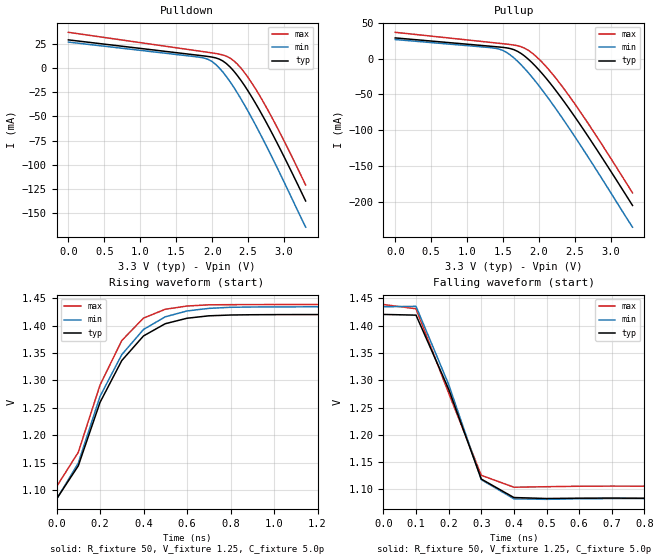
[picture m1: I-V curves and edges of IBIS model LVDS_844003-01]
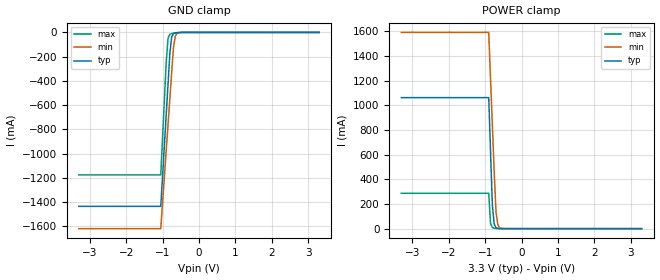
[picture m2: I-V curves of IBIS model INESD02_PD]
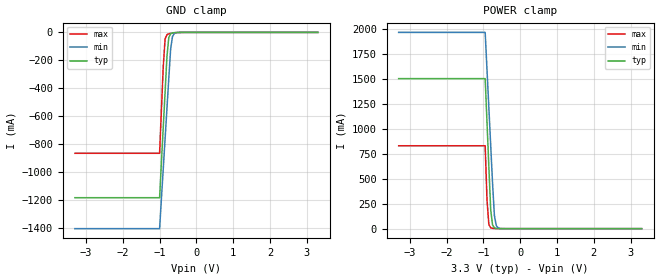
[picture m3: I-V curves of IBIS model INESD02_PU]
|   This file is an IBIS representation of the   |
|   Integrated Device Technology, Inc.   |
|   ICS844003-01   |
[IBIS Ver]   4.0
[File name]   844003-01_3v3.ibs
[File Rev]   1.0
[Date]   Sep 5 2007  | Last modified
|   Sep 5 2007  | Generated
[Source] Originated at Integrated Device Technology, Inc.
[Disclaimer]
IDT hereby grants the user of this IBIS model a non-exclusive,
nontransferable license to use this IBIS model under the following terms.
Before using this IBIS model, the user should read this license.
If the user does not accept these terms,  the IBIS model should be
returned to IDT within 30 days.
   The user is granted this license only to use the IBIS model and
is not granted rights to sell, load, rent, lease or license the IBIS
model in whole or in part, or in modified form to anyone other than
user. User may modify the IBIS model to suit its specific
applications but rights to derivative works and such modifications
shall belong to IDT.
   This IBIS model is provided on an "AS IS" basis and IDT makes
absolutely no warranty with respect to the information contained
herein. IDT DISCLAIMS AND CUSTOMER WAIVES ALL WARRANTIES, EXPRESS
OR IMPLIED, INCLUDING WARRANTIES OF MERCHANTABILITY OR FITNESS FOR
A PARTICULAR PURPOSE. The entire risk as to quality and performance
is with the Customer. ACCORDINGLY, IN NO EVENT SHALL THE COMPANY BE
LIABLE FOR ANY DAMAGES, WHETHER IN CONTRACT OR TORT,INCLUDING ANY
LOST PROFITS OR OTHER INCIDENTAL, CONSEQUENTIAL, EXEMPLARY, OR
PUNITIVE DAMAGES ARISING OUT OF THE USE OR APPLICATION OF THE IBIS
model provided in this package. Further, IDT reserves the right to
make changes without notice to any product herein to improve
reliability, function, or design. IDT does not convey any license
under patent rights or any other intellectual property rights,
including those of third parties.
   IDT is not obligated to provide maintenance or support
for the licensed IBIS model.
[Copyright]   Copyright 2007 by Integrated Device Technology, Inc.
[Component]   ICS844003BG-01
[Manufacturer] Integrated Device Technology, Inc.
[Package]
|TSSOP 24 Lead
|   typ   min   max
R_pkg   60.65m   52.4m   68.9m
L_pkg   1.989nH   1.431nH   2.547nH
C_pkg   0.314pF   0.254pF   0.374pF
[Pin] signal_name  model_name   R_pin   L_pin   C_pin
1   DIV_SELB0   INESD02_PU   68.9m   2.547n   0.374p
2   VCO_SEL   INESD02_PU   65.6m   2.323n   0.350p
3   MR   INESD02_PD   62.3m   2.100n   0.326p
4   VDDO_A   POWER   59.0m   1.877n   0.302p
5   QA0   LVDS_844003-01   55.7m   1.654n   0.278p
6   nQA0   LVDS_844003-01   52.4m   1.431n   0.254p
7   OEB   INESD02_PU   52.4m   1.431n   0.254p
8   OEA   INESD02_PU   55.7m   1.654n   0.278p
9   FB_DIV   INESD02_PD   59.0m   1.877n   0.302p
10   VDDA   POWER   62.3m   2.100n   0.326p
11   VDD   POWER   65.6m   2.323n   0.350p
12   DIV_SELA0   INESD02_PU   68.9m   2.547n   0.374p
13   DIV_SELA1   INESD02_PU   68.9m   2.547n   0.374p
14   GND   GND   65.6m   2.323n   0.350p
|15  XTAL_OUT   62.3m   2.100n   0.326p
|16  XTAL_IN   59.0m   1.877n   0.302p
17   REF_CLK   INESD02_PD   55.7m   1.654n   0.278p
18   XTAL_SEL   INESD02_PU   52.4m   1.431n   0.254p
19   nQB1   LVDS_844003-01   52.4m   1.431n   0.254p
20   QB1   LVDS_844003-01   55.7m   1.654n   0.278p
21   nQB0   LVDS_844003-01   59.0m   1.877n   0.302p
22   QB0   LVDS_844003-01   62.3m   2.100n   0.326p
23   VDDO_B   POWER   65.6m   2.323n   0.350p
24   DIV_SELB1   INESD02_PU   68.9m   2.547n   0.374p
[Diff Pin]  inv_pin  vdiff tdelay_typ tdelay_min  tdelay_max
5   6   NA   0  0  0
20   19   NA   0  0  0
22   21   NA   0  0  0
| Models and submodels in the file (3): LVDS_844003-01 (Output_ECL), INESD02_PD (Input), INESD02_PU (Input)
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[Model]   LVDS_844003-01
Model_type   Output_ECL
Polarity   Non-Inverting
|   onlvds01_lvds03_vrlvds06_abiasoff01_3v3_8402010i
|   typ   min   max
C_comp   2pF   1.5pF   2.5pF
Vmeas = 1.25V
Rref = 50
Vref = 1.25V
|   typ   min   max
[Voltage range]   3.3V   3.135V   3.465V
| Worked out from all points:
|   rising waveform, R_fixture 50, V_fixture 1.25, C_fixture 5.0p: 20-80 % time 231ps typ, 234ps min, 196ps max; typ from 1.08 V to 1.42 V
|   falling waveform, R_fixture 50, V_fixture 1.25, C_fixture 5.0p: 20-80 % time 132ps typ, 130ps min, 131ps max; typ from 1.42 V to 1.08 V
[pulldown]
|Voltage   I (typ)   I (min)   I (max)
0V        29.08mA    26.8mA     36.89mA
1.8V      13.22mA    11.37mA    17.73mA
1.9V      12.32mA    10.03mA    16.66mA
2V        11.24mA    6.613mA    15.58mA
2.15V     7.191mA    -4.325mA   13.43mA
2.25V     965.3uA    -14.33mA   10.19mA
2.35V     -7.741mA   -25.77mA   4.035mA
2.5V      -23.89mA   -44.84mA   -9.868mA
2.65V     -42.52mA   -65.56mA   -27.29mA
2.85V     -69.92mA   -94.93mA   -53.84mA
3.05V     -99.22mA   -125.7mA   -82.8mA
3.3V      -137.5mA   -164.6mA   -121mA
[pullup]
|Voltage   I (typ)   I (min)   I (max)
0V        29.08mA    26.8mA     36.89mA
1.35V     17.18mA    15.14mA    22.52mA
1.5V      15.75mA    11.38mA    20.91mA
1.6V      14.13mA    5.181mA    19.77mA
1.75V     7.285mA    -8.508mA   16.68mA
1.9V      -5.36mA    -25.52mA   8.171mA
2.05V     -21.61mA   -44.7mA    -5.816mA
2.2V      -40.2mA    -65.36mA   -23.15mA
2.4V      -67.42mA   -94.5mA    -49.51mA
2.65V     -104mA     -132.6mA   -85.74mA
2.95V     -150.1mA   -180mA     -132mA
3.3V      -205.5mA   -235.9mA   -187.9mA
[Ramp]
|   typ   min   max
dV/dt_r   0.24/0.3n   0.24/0.35n   0.24/0.25n
dV/dt_f   0.24/0.3n   0.24/0.35n   0.24/0.25n
[Rising Waveform]
R_fixture = 50
V_fixture = 1.25
V_fixture_max = 1.28
V_fixture_min = 1.22
C_fixture = 5.0p
| Time   typ   min   max
0s        1.083V     1.083V     1.106V
100ps     1.144V     1.149V     1.169V
200ps     1.26V      1.271V     1.292V
300ps     1.336V     1.347V     1.373V
400ps     1.381V     1.393V     1.414V
500ps     1.404V     1.416V     1.43V
600ps     1.414V     1.427V     1.436V
800ps     1.42V      1.434V     1.438V
1ns       1.42V      1.435V     1.439V
5ns       1.421V     1.435V     1.439V
[Falling Waveform]
R_fixture = 50
V_fixture = 1.25
V_fixture_max = 1.28
V_fixture_min = 1.22
C_fixture = 5.0p
| Time   typ   min   max
0s        1.421V     1.435V     1.439V
100ps     1.419V     1.435V     1.431V
200ps     1.284V     1.292V     1.277V
300ps     1.119V     1.118V     1.126V
400ps     1.085V     1.083V     1.104V
500ps     1.083V     1.082V     1.105V
700ps     1.084V     1.083V     1.106V
5ns       1.083V     1.083V     1.106V
[Model]   INESD02_PD
Model_type   Input
Polarity   Non-Inverting
Vinl = 0.80V
Vinh = 2.0V
|   typ   min   max
C_comp   2pF   1.5pF   2.5pF
|   typ   min   max
[Voltage range]  3.3V   3.15V   3.45V
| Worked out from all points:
|   GND clamp passes 1 mA (typ) near -0.56 V on its own axis
|   POWER clamp passes 1 mA (typ) near -0.61 V on its own axis
[GND_clamp]
|Voltage   I(typ)   I(min)   I(max)
-3.3V     -1.436A    -1.62A     -1.176A
-1.05V    -1.436A    -1.62A     -1.176A
-900mV    -678.5mA   -975.1mA   -244mA
-850mV    -426.1mA   -760.1mA   -46.85mA
-800mV    -173.9mA   -545.4mA   -16.11mA
-750mV    -36.96mA   -330.7mA   -9.916mA
-700mV    -9.696mA   -120.2mA   -7.056mA
-650mV    -3.545mA   -29.7mA    -4.857mA
-600mV    -1.629mA   -7.52mA    -3.049mA
-400mV    -52.81uA   -52.52uA   -108.7uA
3.3V      71.13uA    77.43uA    62.11uA
[POWER_clamp]
|Voltage   I(typ)   I(min)   I(max)
-3.3V     1.063A     1.593A     287.3mA
-900mV    1.063A     1.593A     287.3mA
-850mV    620.5mA    1.215A     41.84mA
-800mV    191.6mA    837.5mA    8.757mA
-750mV    37.76mA    460.2mA    3.328mA
-700mV    8.104mA    133.8mA    1.728mA
-650mV    2.076mA    32.66mA    905.3uA
-600mV    678.1uA    8.083mA    443.8uA
-450mV    104.2uA    213.3uA    89.09uA
3.3V      -3.041nA   -3.986uA   0A
[Model]   INESD02_PU
Model_type   Input
Polarity   Non-Inverting
Vinl = 0.80V
Vinh = 2.0V
|   typ   min   max
C_comp   2pF   1.5pF   2.5pF
|   typ   min   max
[Voltage range]  3.3V   3.15V   3.45V
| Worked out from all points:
|   GND clamp passes 1 mA (typ) near -0.56 V on its own axis
|   POWER clamp passes 1 mA (typ) near -0.61 V on its own axis
[GND_clamp]
|Voltage   I(typ)   I(min)   I(max)
-3.3V     -1.184A    -1.405A    -865.6mA
-1V       -1.184A    -1.405A    -865.6mA
-900mV    -678.5mA   -975.1mA   -244.1mA
-850mV    -426.2mA   -760.2mA   -46.92mA
-800mV    -174mA     -545.4mA   -16.17mA
-750mV    -37.03mA   -330.8mA   -9.981mA
-700mV    -9.767mA   -120.3mA   -7.122mA
-650mV    -3.616mA   -29.78mA   -4.922mA
-600mV    -1.7mA     -7.594mA   -3.115mA
-400mV    -123.9uA   -126uA     -173.9uA
3.3V      1.866nA    3.949uA    0A
[POWER_clamp]
|Voltage   I(typ)   I(min)   I(max)
-3.3V     1.506A     1.97A      832.1mA
-950mV    1.506A     1.97A      832.1mA
-900mV    1.063A     1.592A     287.2mA
-850mV    620.4mA    1.215A     41.77mA
-800mV    191.5mA    837.4mA    8.692mA
-750mV    37.69mA    460.1mA    3.262mA
-700mV    8.032mA    133.8mA    1.662mA
-650mV    2.005mA    32.58mA    840.1uA
-600mV    607uA      8.009mA    378.6uA
-450mV    33.11uA    139.8uA    23.88uA
3.3V      -71.13uA   -77.46uA   -62.11uA
